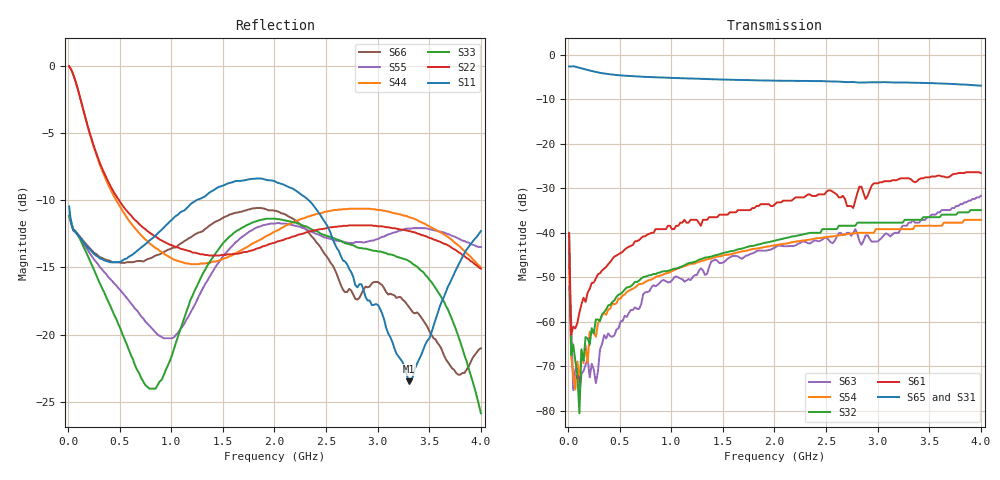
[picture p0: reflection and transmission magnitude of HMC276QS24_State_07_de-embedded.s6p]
! Hittite Microwave Corporation
! 20 Alpha Road
! Chelmsford, MA 01824
! Tel: 978-250-3343
! Fax: 978-250-3373
! Device: HMC276QS24, 0.7-3.0 GHz, GaAS MMIC 4x2 Switch Matrix in 24-lead QSOP package
! Misc: Data was de-embedded to package pins.
!  Port 1 = OP1
!  Port 2 = VL
!  Port 3 = VH
!  Port 4 = HH
!  Port 5 = HL
!  Port 6 = OP2
!  Vdd = +5 V
!  Vctl = 0 V[Logic 0] / +5 V[Logic 1]
!  State 07,  VH to OP1,  HL to OP2
!  Control Lines (Logic)
!  HV 1 = 0, Tone 1 = 1
!  HV 2 = 1, Tone 2 = 0
!  Data reformated to new Touchstone file format - Wed Jan 10 15:15:55 2007
# MHz S DB R 50
! 6 Port Network Data
! freq  dbS11  angS11  dbS12  angS12  dbS13  angS13  dbS14  angS14
!  dbS15  angS15  dbS16  angS16
!  dbS21  angS21  dbS22  angS22
!  dbS23  angS23  dbS24  angS24  dbS25  angS25  dbS26  angS26
!  dbS31  angS31  dbS32  angS32  dbS33  angS33  dbS34  angS34
!  dbS35  angS35  dbS36  angS36
!  dbS41  angS41  dbS42  angS42
!  dbS43  angS43  dbS44  angS44  dbS45  angS45  dbS46  angS46
!  dbS51  angS51  dbS52  angS52  dbS53  angS53  dbS54  angS54
!  dbS55  angS55  dbS56  angS56
!  dbS61  angS61  dbS62  angS62
!  dbS63  angS63  dbS64  angS64  dbS65  angS65  dbS66  angS66
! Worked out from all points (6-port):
!   201 points, 10 MHz to 4 GHz, reference 50 ohm
!   strongest paths, dB at 10 MHz, 1.008 GHz, 2.005 GHz, 3.002 GHz, 4 GHz:
!     S65: -2.6, -5.2, -5.8, -6.2, -6.9
!     S31: -2.7, -5.4, -6.1, -6.1, -7.0
!     S61: -40.2, -39.2, -33.6, -28.9, -26.6
!     S32: -40.0, -48.3, -41.7, -37.7, -34.9
!     S54: -46.9, -48.6, -42.8, -39.2, -37.1
!     S63: -52.1, -50.7, -43.3, -41.9, -31.7
!   lowest |S11| = -23.5 dB at 3.302 GHz (marker M1), VSWR 1.14, Z = 56.3 + j3.35 ohm
!   |S11| at or under -10 dB: start of sweep to 1.243 GHz; 2.331 GHz to end of sweep
